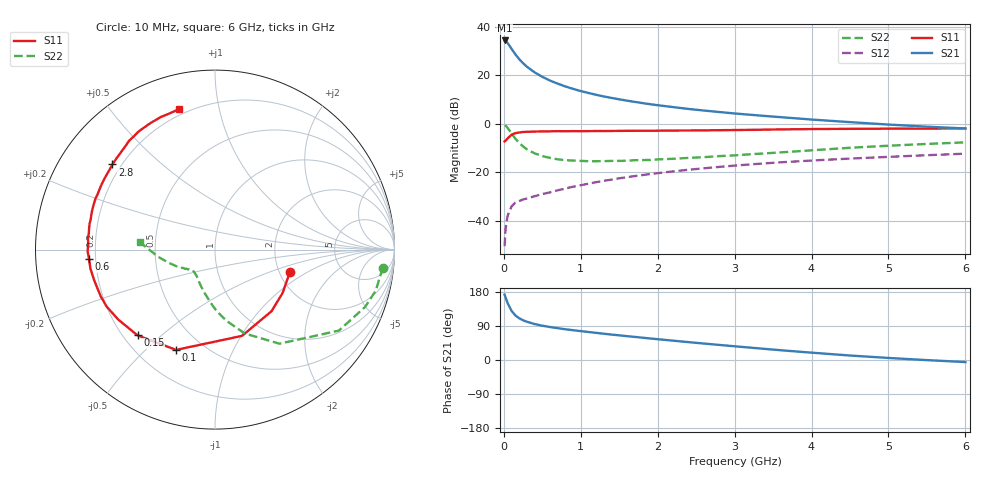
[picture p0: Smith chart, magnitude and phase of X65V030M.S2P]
! SIEMENS Small Signal Semiconductors
! BFP193W
! Si NPN RF Bipolar Junction Transistor in SOT343
! VCE = 5 V  IC = 30 mA
! Common Emitter S-Parameters:  April 1994
# GHz  S  MA  R  50
!  f  S11  S21  S12  S22
! GHz  MAG  ANG  MAG  ANG  MAG  ANG  MAG  ANG
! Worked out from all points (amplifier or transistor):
!   40 points, 10 MHz to 6 GHz, reference 50 ohm
!   highest |S21| = 34.5 dB at 10 MHz (marker M1)
!   |S21| within 3 dB of that: start of sweep to 90.51 MHz
!   unconditionally stable (mu >= 1): 808.1 MHz to 3.969 GHz
!   at 200 MHz: K = 0.44, MSG = 29.3 dB, |S12| = -31.8 dB
!   at 1.5 GHz: K = 1.11, MAG = 14.3 dB, |S12| = -22.4 dB
!   at 6 GHz: K = 0.93, MSG = 5.2 dB, |S12| = -12.3 dB
!   lowest NFmin = 1.90 dB at 450 MHz
!   S11 on the Smith chart (normalised r, x): 10 MHz: 2.29, -0.70; 100 MHz: 0.36, -0.62; 150 MHz: 0.26, -0.42; 600 MHz: 0.17, -0.04; 2.8 GHz: 0.17, +0.35; 6 GHz: 0.17, +0.76
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0.01  0.4357 -16.4  52.8 172.4  0.003 88.8  0.9398 -6.2
0.02  0.4476 -32.7  52.03 166.8  0.006 77.1  0.9246 -14.3
0.03  0.4658 -47.4  50.69 160.8  0.0085 75.5  0.8953 -20.9
0.05  0.5037 -72.6  46.49 149.6  0.0129 65.7  0.8244 -33.2
0.1  0.5993 -111.2  35.52 129.9  0.0198 51.1  0.6354 -55.6
0.15  0.644 -132.1  27.3 117.6  0.0239 44.6  0.4955 -70.5
0.2  0.6651 -144.1  21.66 110.1  0.0256 42.7  0.4036 -80.6
0.25  0.682 -152.2  17.95 104.8  0.0276 41.5  0.3441 -88.3
0.3  0.6878 -157.7  15.15 100.9  0.0289 42.1  0.2983 -94.5
0.4  0.6946 -165.8  11.61 94.9  0.0322 44.3  0.2469 -103.9
0.5  0.7022 -171.4  9.382 90.5  0.0357 47.0  0.2171 -111.3
0.6  0.7038 -175.7  7.843 87.0  0.0387 49.3  0.1985 -117.0
0.8  0.7067 177.7  5.934 81.1  0.0464 52.9  0.179 -124.8
1.1  0.7112 170.6  4.358 73.9  0.0584 56.0  0.1702 -132.6
1.3  0.7126 166.2  3.69 69.3  0.067 57.1  0.1711 -135.6
1.6  0.7202 160.4  3.025 62.9  0.0796 57.6  0.1742 -139.2
2.2  0.7289 150.0  2.226 51.0  0.1049 55.9  0.1908 -145.9
2.8  0.7425 140.3  1.761 39.8  0.1298 52.8  0.2165 -152.1
3.2  0.7535 134.3  1.548 32.7  0.1459 50.1  0.2363 -157.1
4.5  0.7914 117.0  1.089 11.8  0.1926 41.2  0.3222 -173.2
5.5  0.8 108.4  0.877 -0.3  0.2261 34.8  0.3863 177.8
6  0.8082 104.2  0.806 -5.5  0.2434 32.0  0.417 174.5
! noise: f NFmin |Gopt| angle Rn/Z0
0.45  1.9  0.4  180  0.09
0.9  1.95  0.43  -173  0.11
1.8  2.4  0.58  -144  0.24
